(*此PLC项目为FB_XmlSrvRead对应例程,FB_XmlSrvWrite请打开名称为XML Server的PLC项目*)
PROGRAM MAIN
VAR
	ST_XmlWrite1: ST_XmlTest1;
	FB_XmlRead: FB_XmlSrvRead;
	b_Execute: BOOL;
	sFilePath: T_MaxString:='Hard Disk\temp\Test.xml';		
	sXPath: T_MaxString:='/dataentry/MAIN.ST_XmlWrite1';
END_VAR

FB_XmlRead(
	sNetId:= , 							//默认为本地的NetId,连接控制器后使用的是控制器本地的编程环境，也可以不填写
	ePath:= PATH_GENERIC, 				//用于在目标设备上选择用于打开文件的TwinCAT系统路径,PATH_GENERIC即表示在选定/通用文件夹中搜索/打开/创建文件
	nMode:= XMLSRV_ADDMISSING, 			//用于控制XML文件的计算方式,具体解释可参考文档说明
	pSymAddr:= ADR(ST_XmlWrite1), 		//将XML文件中的数据读取到PLC变量的地址
	cbSymSize:= SIZEOF(ST_XmlWrite1), 	//将XML文件中的数据读取到PLC变量的大小
	sFilePath:= sFilePath, 				
	sXPath:= sXPath, 
	bExecute:= b_Execute, 				//功能块触发条件，置TRUE则执行一次
	tTimeout:= , 						//功能块执行的最大时间，超时报错
	bBusy=> , 
	bError=> , 
	nErrId=> );

END_PROGRAM
